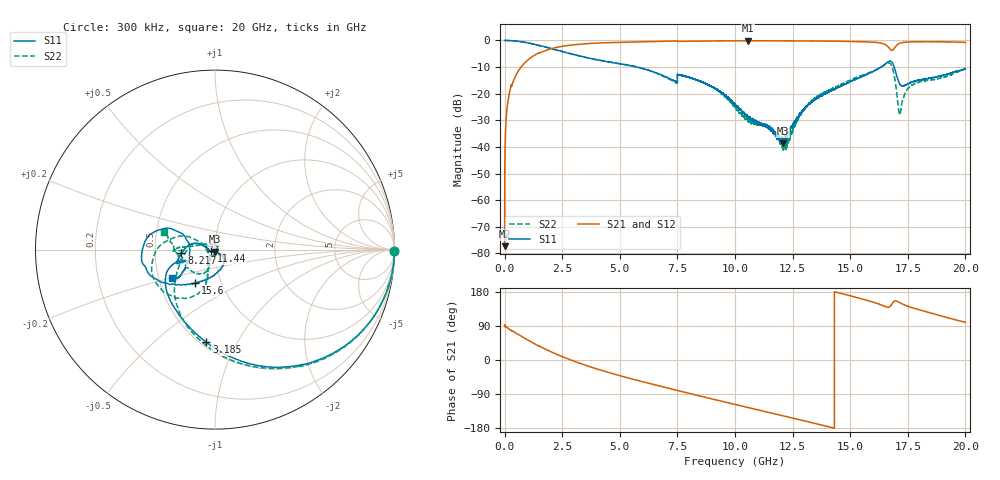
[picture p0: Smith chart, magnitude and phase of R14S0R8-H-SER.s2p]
!{R14S0R8}
!Johanson Technology Inc.
!www.johansontechnology.com
!Test Board Conditions:
!Substrate Type  RO4350B
!Substrate Thickness  20 mil
!Substrate Dk  3.66
!TL Type: GCPW
!TL Trace Width  36 mil
!TL Gap  12 mil
!Electrode orientation  Horizontal
!DUT TOPOLOGY	SERIES
!Mounting Pad LxW  26x36 mil
! Created Wed Nov 25 17:33:21 2020
! 2 Port Network Data from SP1.SP block
! freq  magS11  angS11  magS21  angS21  magS12  angS12  magS22  angS22
# khz S ma R 50
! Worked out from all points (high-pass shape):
!   20001 points, 300 kHz to 20 GHz, reference 50 ohm
!   highest |S21| = -0.11 dB at 10.58 GHz (marker M1); lowest = -77.3 dB at 300 kHz (marker M2)
!   |S21| within 3 dB of the highest: 2.03 GHz to 16.72 GHz (14.69 GHz wide, 157 % of centre); 16.9 GHz to end of sweep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
!   lowest |S11| = -38.6 dB at 12.08 GHz (marker M3), VSWR 1.02, Z = 49.8 - j1.17 ohm
!   |S11| at or under -10 dB: 5.73 GHz to 16.34 GHz (10.61 GHz wide, 96.1 % of centre); 16.91 GHz to end of sweep
!   |S22| runs from -41.3 to 0.0 dB; largest |S21 - S12| = 0.015
!   S11 on the Smith chart (normalised r, x): 300 kHz: open; 3.185 GHz: 0.54, -0.76; 8.217 GHz: 0.68, -0.03; 11.44 GHz: 0.96, -0.02; 15.6 GHz: 0.75, -0.29; 20 GHz: 0.58, -0.20
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300  0.9999 -0.3  0.0001367 93.0  0.0001386 90.2  0.9999 -0.3
101300  0.9979 -4.2  0.05104 85.5  0.05128 85.6  0.9986 -4.2
132300  0.9974 -5.4  0.06653 84.2  0.06684 84.3  0.9974 -5.4
255300  0.9906 -10.6  0.1276 78.9  0.1281 78.8  0.9904 -10.6
496300  0.9732 -18.6  0.2237 70.9  0.2242 71.0  0.9719 -18.7
1500300  0.8073 -52.3  0.578 37.0  0.579 36.9  0.806 -53.3
3185300  0.5187 -95.3  0.8434 -6.8  0.8446 -6.9  0.5191 -98.2
3334300  0.5008 -98.6  0.8546 -10.0  0.8556 -10.1  0.5011 -101.3
5077300  0.3596 -137.6  0.9232 -42.6  0.9238 -42.6  0.3614 -127.3
6667300  0.2382 -161.2  0.9611 -67.8  0.9609 -67.7  0.2353 -151.9
8217300  0.1881 -173.7  0.9681 -91.3  0.9712 -91.1  0.1888 175.6
1.00003e7  0.06469 161.6  0.9843 -117.2  0.9831 -117.2  0.05624 147.6
1.05783e7  0.03445 179.4  0.9878 -125.6  0.9834 -125.5  0.02961 104.1
1.14393e7  0.02356 -155.4  0.9842 -137.9  0.9843 -138.0  0.02364 56.6
1.20823e7  0.0118 -97.4  0.9839 -147.2  0.9841 -147.2  0.01023 -7.2
1.33343e7  0.07092 -45.8  0.9768 -165.3  0.98 -165.3  0.07408 -114.2
1.55963e7  0.2164 -121.1  0.9442 159.8  0.9459 159.8  0.2273 -106.5
1.66673e7  0.3996 -165.7  0.7411 139.2  0.7319 139.6  0.3765 -149.7
1.68643e7  0.3578 164.8  0.6677 152.6  0.6628 153.2  0.2772 170.5
1.71573e7  0.1501 165.6  0.8878 151.0  0.8879 151.4  0.04225 -143.4
1.77173e7  0.1673 -156.7  0.9417 137.4  0.9403 137.3  0.1467 -116.4
2e7  0.2895 -146.8  0.9188 99.3  0.9103 99.2  0.3013 160.6
